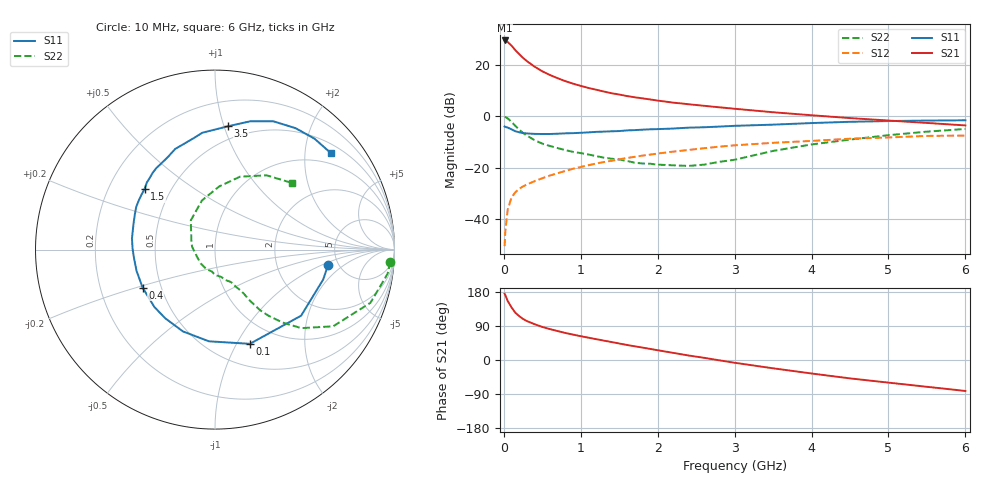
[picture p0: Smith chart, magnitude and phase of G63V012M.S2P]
! SIEMENS Small Signal Semiconductors
! BFG193
! Si NPN RF Bipolar Junction Transistor in SOT223
! VCE = 3 V  IC = 12 mA
! Common Emitter S-Parameters:  August  1996
# GHz  S  MA  R  50
!  f  S11  S21  S12  S22
! GHz  MAG  ANG  MAG  ANG  MAG  ANG  MAG  ANG
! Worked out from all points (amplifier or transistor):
!   36 points, 10 MHz to 6 GHz, reference 50 ohm
!   highest |S21| = 29.7 dB at 10 MHz (marker M1)
!   |S21| within 3 dB of that: start of sweep to 127.1 MHz
!   unconditionally stable (mu >= 1): 818.8 MHz to 2.581 GHz
!   at 250 MHz: K = 0.60, MSG = 25.1 dB, |S12| = -27.4 dB
!   at 1.4 GHz: K = 1.06, MAG = 11.7 dB, |S12| = -17.3 dB
!   at 6 GHz: K = 0.88, MSG = 2.0 dB, |S12| = -7.5 dB
!   S11 on the Smith chart (normalised r, x): 10 MHz: 4.13, -1.20; 100 MHz: 0.74, -1.14; 400 MHz: 0.39, -0.21; 1.5 GHz: 0.36, +0.33; 3.5 GHz: 0.39, +1.03; 6 GHz: 0.71, +2.59
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0.01  0.6359 -7.8  30.62 174.8  0.0029 91.3  0.9793 -4.0
0.02  0.6253 -15.5  30.3 170.6  0.0059 80.5  0.9708 -8.0
0.05  0.6048 -37.5  28.58 155.9  0.0151 73.5  0.9152 -18.9
0.1  0.5597 -69.7  24.2 138.8  0.026 64.4  0.7848 -33.0
0.15  0.5121 -93.8  19.77 124.6  0.0329 56.0  0.6501 -42.3
0.2  0.4896 -111.4  16.55 115.7  0.0385 54.2  0.5539 -47.2
0.25  0.4726 -125.8  13.97 108.3  0.0428 52.2  0.474 -51.0
0.3  0.4651 -136.6  12.06 102.7  0.0467 52.0  0.422 -53.3
0.4  0.4555 -152.3  9.399 94.4  0.0541 52.3  0.3425 -55.7
0.5  0.4529 -164.8  7.624 87.2  0.0618 52.6  0.2939 -56.8
0.6  0.4534 -173.4  6.458 81.5  0.0699 53.3  0.2642 -58.3
0.7  0.4592 179.5  5.586 76.3  0.0776 53.4  0.2404 -60.4
0.9  0.4711 166.1  4.378 67.0  0.0948 52.2  0.2027 -63.6
1.1  0.4876 156.4  3.61 58.9  0.1109 50.8  0.1802 -70.7
1.5  0.5173 139.4  2.683 43.6  0.1447 45.4  0.1434 -87.9
1.7  0.5396 132.5  2.371 36.2  0.1621 42.6  0.1244 -97.2
2.2  0.5794 116.8  1.864 18.9  0.205 32.9  0.1108 -135.7
2.8  0.6326 100.7  1.509 -0.8  0.2564 20.6  0.1293 172.4
3.5  0.6908 84.0  1.207 -21.9  0.3048 4.2  0.2116 129.5
4.5  0.7854 65.5  0.928 -48.5  0.3663 -15.6  0.3527 86.2
5.5  0.8302 48.1  0.746 -70.7  0.4161 -39.4  0.5039 55.2
6  0.8401 39.8  0.667 -81.7  0.4228 -53.2  0.5685 40.7
